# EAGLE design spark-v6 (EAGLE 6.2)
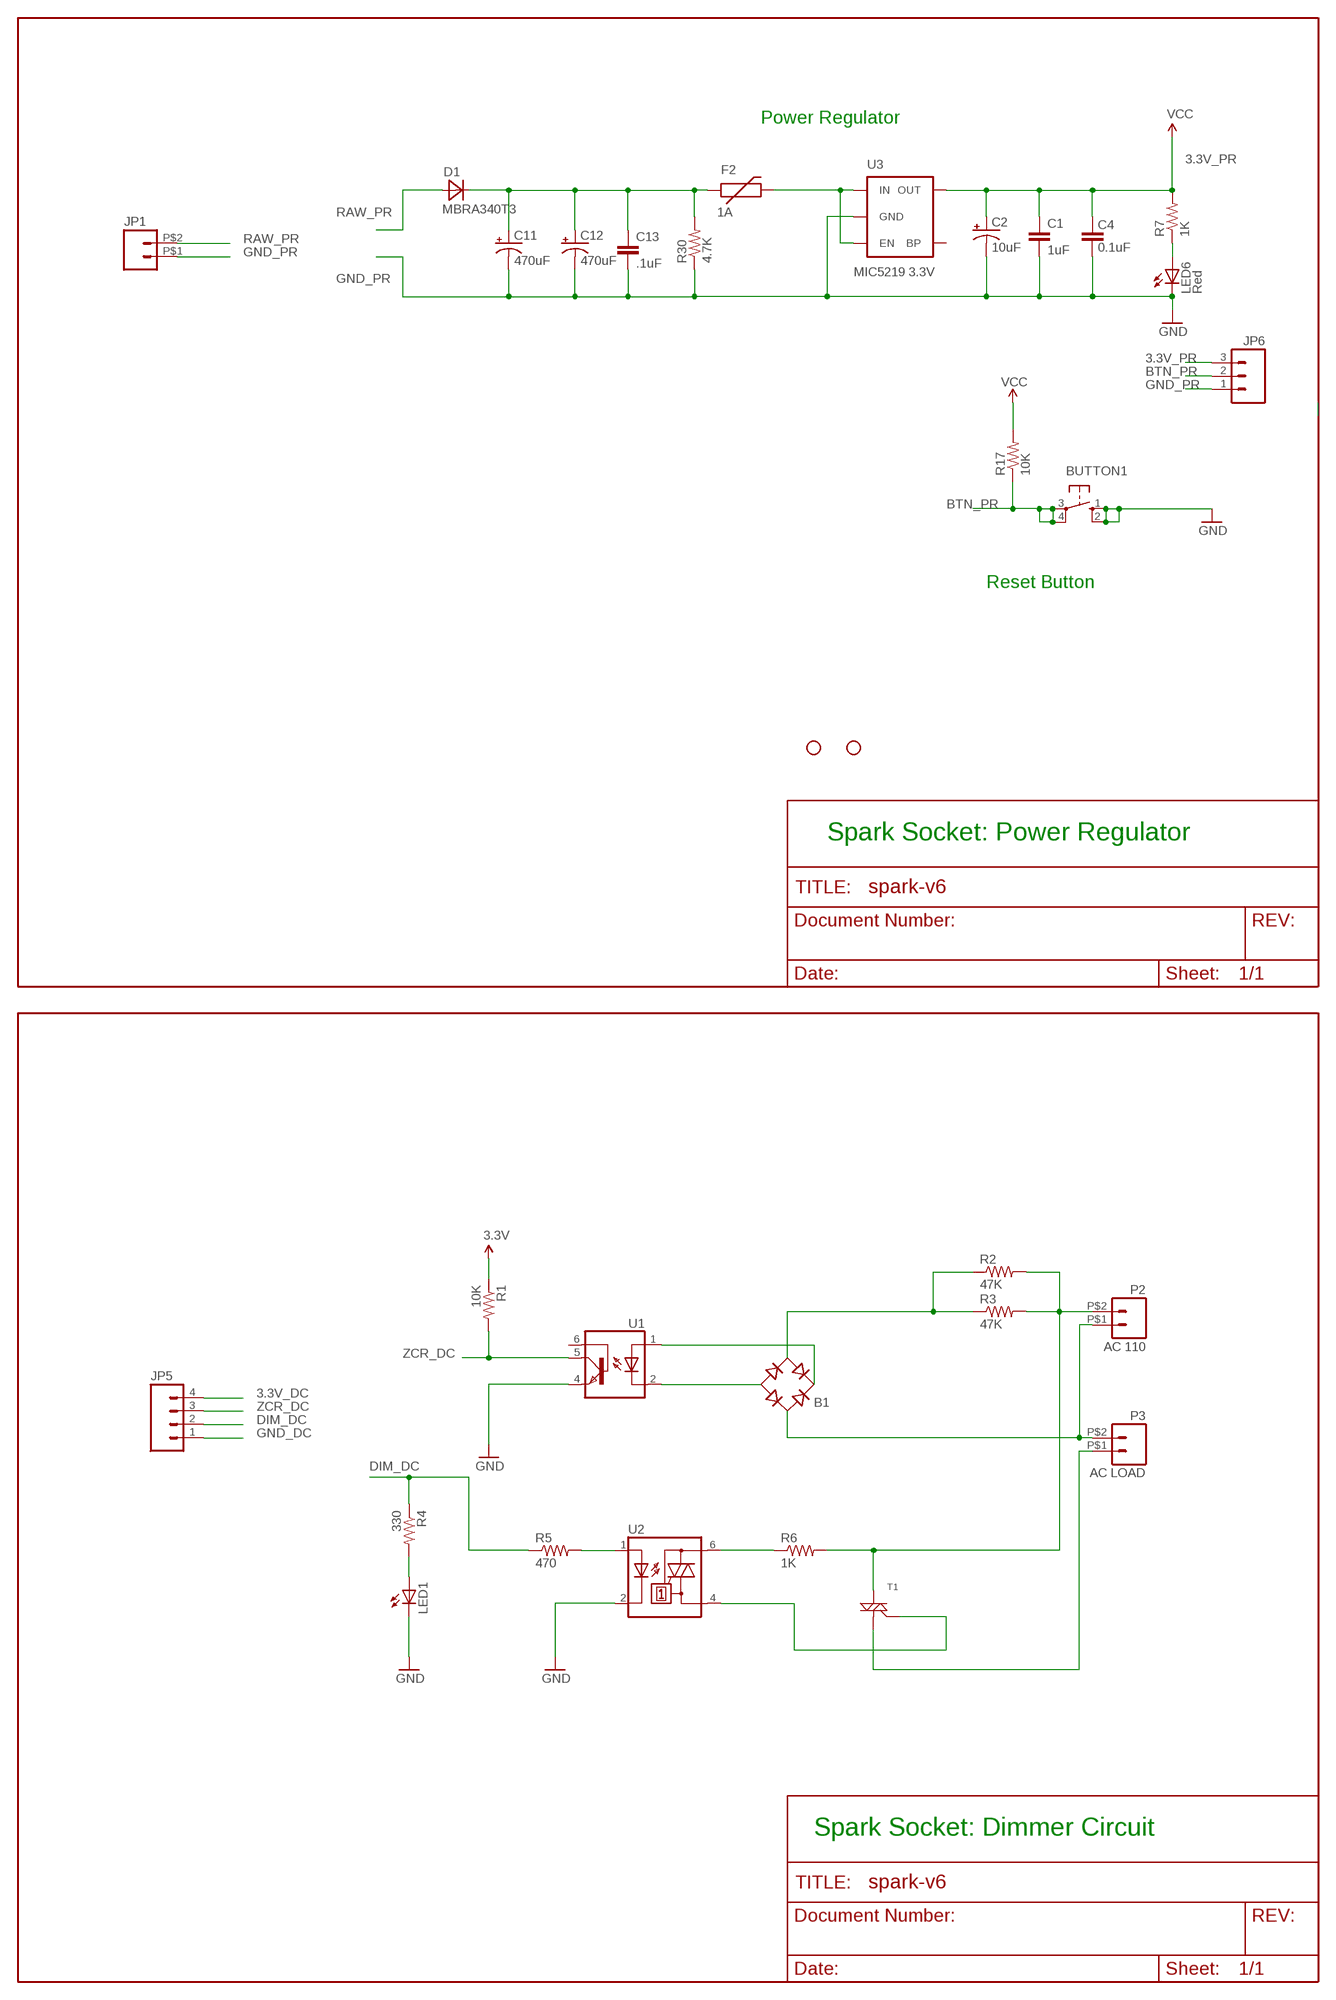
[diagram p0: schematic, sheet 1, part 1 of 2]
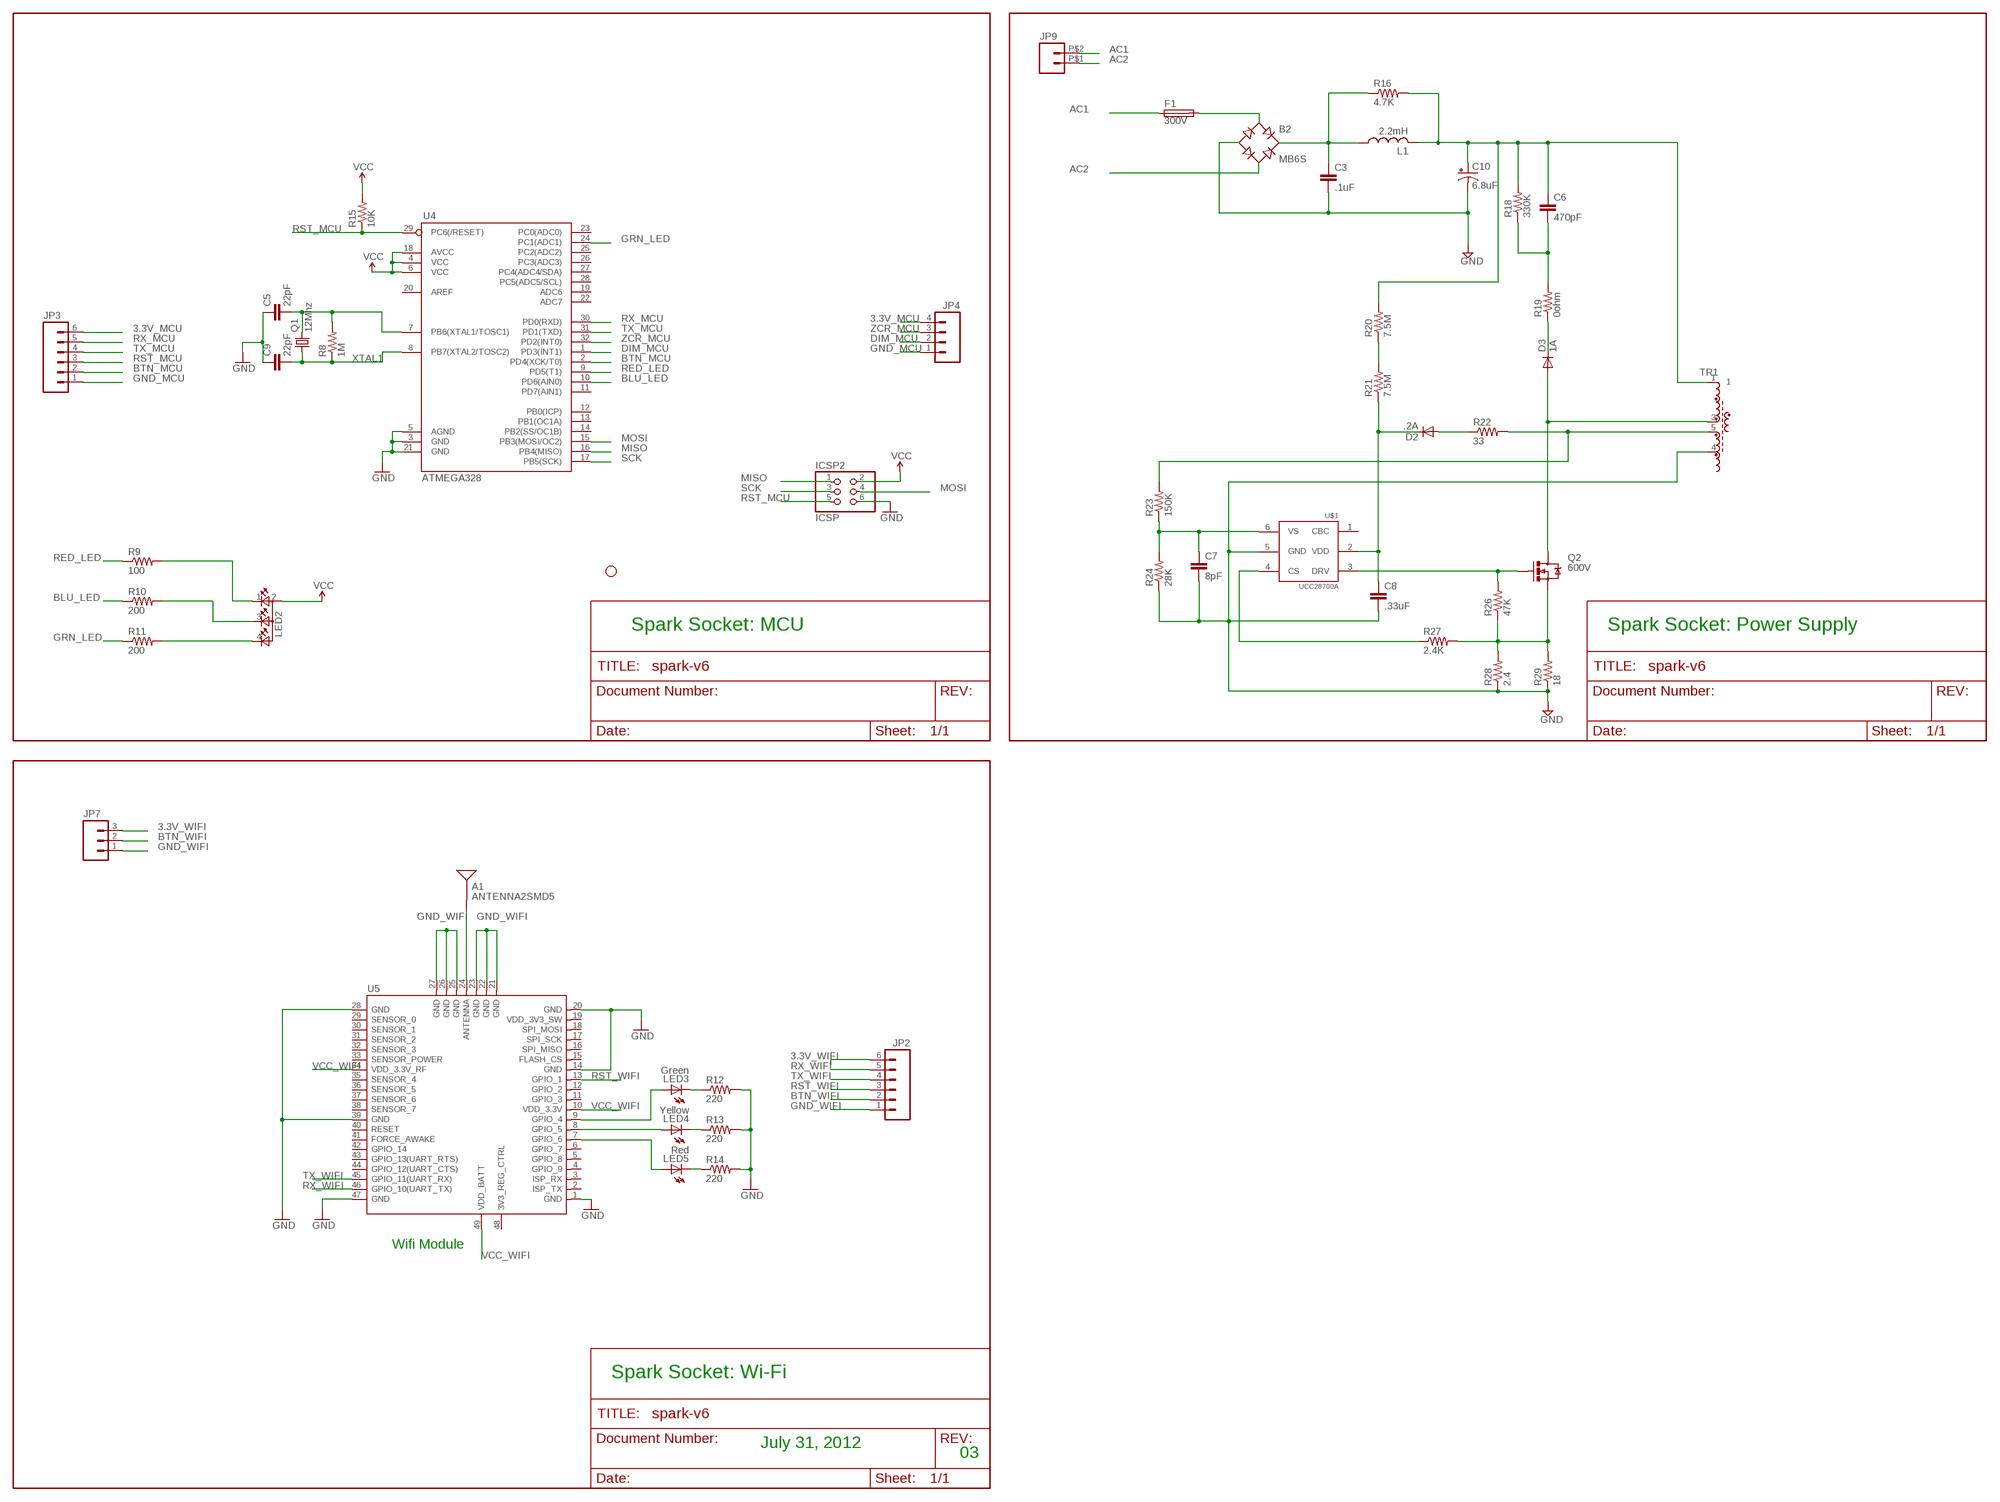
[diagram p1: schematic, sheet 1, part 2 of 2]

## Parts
A1  ANTENNA2SMD5  [ANTENNA-CHIP5]
B1  DF10S  [DFS]
B2  MB6S  [SOIC-4]
BUTTON1  10-XX  [B3F-10XX]
C1  1uF  CAP0603-CAP  [0603-CAP]
C2  10uF  CAP_POL1206  [EIA3216]
C3  .1uF  CAP1206  [1206]
C4  0.1uF  CAP0603-CAP  [0603-CAP]
C5  22pF  CAP0603-CAP  [0603-CAP]
C6  470pF  CAP1206  [1206]
C7  8pF  CAP0603-CAP  [0603-CAP]
C8  .33uF  CAP0603-CAP  [0603-CAP]
C9  22pF  CAP0603-CAP  [0603-CAP]
C10  6.8uF  CPOL-USE5-8.5  [E5-8,5]
C11  470uF  CAP_POL1206  [EIA3216]
C12  470uF  CAP_POL1206  [EIA3216]
C13  .1uF  CAP1206  [1206]
D1  MBRA340T3  [SMA]
D2  .2A  DIODESOD  [SOD-323]
D3  1A  DIODESMA  [SMA-DIODE]
F1  300V  TE5  [TE5]
F2  1A  PTCSMD  [PTC-1206]
ICSP2  ICSP  PINHD-2X3  [2X03]
JP1  M02PTH2  [1X02_BIG]
JP2  M06SIP  [1X06]
JP3  M06SIP  [1X06]
JP4  M04PTH  [1X04]
JP5  M04PTH  [1X04]
JP6  M03PTH  [1X03]
JP7  M03PTH  [1X03]
JP8  STAND-OFF  [STAND-OFF]
JP9  M02PTH2  [1X02_BIG]
JP10  STAND-OFF  [STAND-OFF]
JP11  STAND-OFF  [STAND-OFF]
L1  2.2mH  L-US0204V  [0204V]
LED1  LED0603  [LED-0603]
LED2  TOPLED-3PLCC  [P-LCC-4-3]
LED3  Green  LED0603  [LED-0603]
LED4  Yellow  LED0603  [LED-0603]
LED5  Red  LED0603  [LED-0603]
LED6  Red  LED0603  [LED-0603]
P2  AC 110  M02PTH2  [1X02_BIG]
P3  AC LOAD  M02PTH2  [1X02_BIG]
Q1  12Mhz  CRYSTALHC49UP  [HC49UP]
Q2  600V  MOSFET-NCHANNELPTH2  [TO220V]
R1  10K  RESISTOR0603-RES  [0603-RES]
R2  47K  RESISTOR0603-RES  [0603-RES]
R3  47K  RESISTOR0603-RES  [0603-RES]
R4  330  RESISTOR0603-RES  [0603-RES]
R5  470  RESISTOR0603-RES  [0603-RES]
R6  1K  RESISTOR0603-RES  [0603-RES]
R7  1K  RESISTOR0603-RES  [0603-RES]
R8  1M  RESISTOR0603-RES  [0603-RES]
R9  100  RESISTOR0603-RES  [0603-RES]
R10  200  RESISTOR0603-RES  [0603-RES]
R11  200  RESISTOR0603-RES  [0603-RES]
R12  220  RESISTOR0603-RES  [0603-RES]
R13  220  RESISTOR0603-RES  [0603-RES]
R14  220  RESISTOR0603-RES  [0603-RES]
R15  10K  RESISTOR0603-RES  [0603-RES]
R16  4.7K  RESISTOR0805-RES  [0805]
R17  10K  RESISTOR0603-RES  [0603-RES]
R18  330K  RESISTOR1206  [1206]
R19  0ohm  RESISTOR1206  [1206]
R20  7.5M  RESISTOR1206  [1206]
R21  7.5M  RESISTOR1206  [1206]
R22  33  RESISTOR0603-RES  [0603-RES]
R23  150K  RESISTOR0603-RES  [0603-RES]
R24  28K  RESISTOR0603-RES  [0603-RES]
R26  47K  RESISTOR0603-RES  [0603-RES]
R27  2.4K  RESISTOR0603-RES  [0603-RES]
R28  2.4  RESISTOR0603-RES  [0603-RES]
R29  18  RESISTOR0805-RES  [0805]
R30  4.7K  RESISTOR0603-RES  [0603-RES]
T1  TRIACSMD  [SOT223]
TR1  EMC13  [EMC13]
U1  4N25SM  [DIL6-SMD]
U2  MOC3031S  [DIL6-SMD]
U3  MIC5219 3.3V  V_REG_LDOSMD  [SOT23-5]
U4  ATMEGA328  ATMEGA168  [TQFP32-08]
U5  WIFI-RN-171  [49P-1.27-26.67X17.78]
U$1  UCC28700A  [DBV]

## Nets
3.3V_DC: JP5.4 R1.1 ; supply symbol labelled 3.3V
3.3V_MCU: ICSP2.2 JP3.6 JP4.4 LED2.2(A2) R15.2 U4.4(VCC) U4.6(VCC) U4.18(AVCC) ; supply symbol labelled VCC
3.3V_PR: C1.1 C2.A(+) C4.2 JP6.3 R7.2 R17.2 U3.5(OUT) ; supply symbol labelled VCC
3.3V_WIFI: JP2.6 JP7.3
AC1: F1.1 JP9.P$2
AC2: B2.~2(AC2) JP9.P$1
ASDF: C11.A(+) C12.A(+) C13.1 D1.C F2.1 R30.2
BLU_LED: R10.1 U4.10(PD6(AIN0))
BTN_MCU: JP3.2 U4.2(PD4(XCK/T0))
BTN_PR: BUTTON1.3(P) BUTTON1.4(P1) JP6.2 R17.1
BTN_WIFI: JP2.2 JP7.2
DIM_DC: JP5.2 R4.1 R5.1
DIM_MCU: JP4.2 U4.1(PD3(INT1))
GND: C7.2 C8.2 R24.1 R28.1 R29.1 TR1.4 U$1.5(GND)
GND_DC: JP5.1 LED1.C U1.4(EMI) U2.2(C) ; supply symbol labelled GND
GND_MCU: C5.1 C9.1 ICSP2.6 JP3.1 JP4.1 U4.3(GND) U4.5(AGND) U4.21(GND) ; supply symbol labelled GND
GND_POWER: B2.- C3.2 C10.- ; supply symbol labelled GND
GND_PR: BUTTON1.1(S) BUTTON1.2(S1) C1.2 C2.C(-) C4.1 C11.C(-) C12.C(-) C13.2 JP1.P$1 JP6.1 LED6.C R30.1 U3.2(GND) ; supply symbol labelled GND
GND_WIFI: JP2.1 JP7.1 R12.2 R13.2 R14.2 U5.1(GND) U5.14(GND) U5.20(GND) U5.21(GND) U5.22(GND) U5.23(GND) U5.25(GND) U5.26(GND) U5.27(GND) U5.28(GND) U5.39(GND) U5.47(GND) ; supply symbol labelled GND
GRN_LED: R11.1 U4.24(PC1(ADC1))
MISO: ICSP2.1 U4.16(PB4(MISO))
MOSI: ICSP2.4 U4.15(PB3(MOSI/OC2))
N$1: LED2.1(CRED) R9.2
N$2: LED6.A R7.1
N$3: F2.2 U3.1(IN) U3.3(EN)
N$4: B1.- U1.2(C)
N$5: B1.+ U1.1(A)
N$6: B1.AC2 R2.1 R3.1
N$7: P2.P$2 R2.2 R3.2 R6.2 T1.2(M2)
N$8: LED2.4(CGREEN) R11.2
N$9: R6.1 U2.6(A2)
N$10: T1.3(G) U2.4(A1)
N$11: P3.P$1 T1.1(M1)
N$12: B1.AC1 P2.P$1 P3.P$2
N$13: LED1.A R4.2
N$15: LED2.3(CBLUE) R10.2
N$16: R5.2 U2.1(A)
N$18: B2.~1(AC1) F1.2
N$19: LED3.A U5.9(GPIO_4)
N$20: LED3.C R12.1
N$21: LED4.C R13.1
N$22: LED5.C R14.1
N$23: LED4.A U5.8(GPIO_5)
N$24: LED5.A U5.7(GPIO_6)
N$25: A1.FEED(SIGNAL) U5.24(ANTENNA)
N$26: R20.1 R21.2
N$27: B2.+ C3.1 L1.1 R16.1
N$28: C6.1 C10.+ L1.2 R16.2 R18.2 R20.2 TR1.1
N$29: C6.2 R18.1 R19.2
N$30: D3.A Q2.2(D) TR1.3
N$31: C7.1 R23.1 R24.2 U$1.6(VS)
N$32: D3.C R19.1
N$34: D2.2(A) R22.1
N$35: R22.2 R23.2 TR1.5
N$36: C8.1 D2.1(C) R21.1 U$1.2(VDD)
N$37: R27.1 U$1.4(CS)
N$38: C5.2 Q1.2 R8.2 U4.7(PB6(XTAL1/TOSC1))
N$39: Q2.1(G) R26.2 U$1.3(DRV)
N$40: Q2.3(S) R26.1 R27.2 R28.2 R29.2
RAW_PR: D1.A JP1.P$2
RED_LED: R9.1 U4.9(PD5(T1))
RST_MCU: ICSP2.5 JP3.3 R15.1
RST_WIFI: JP2.3 U5.13(GPIO_1)
RX_MCU: JP3.5 U4.30(PD0(RXD))
RX_WIFI: JP2.5 U5.46(GPIO_10(UART_TX))
SCK: ICSP2.3 U4.17(PB5(SCK))
TX_MCU: JP3.4 U4.31(PD1(TXD))
TX_WIFI: JP2.4 U5.45(GPIO_11(UART_RX))
VCC_WIFI: U5.10(VDD_3.3V) U5.34(VDD_3.3V_RF) U5.49(VDD_BATT)
XTAL1: C9.2 Q1.1 R8.1
ZCR_DC: JP5.3 R1.2 U1.5(COL)
ZCR_MCU: JP4.3 U4.32(PD2(INT0))
Unconnected: U1.6(BAS) U3.4(BP) U4.8(PB7(XTAL2/TOSC2)) U4.11(PD7(AIN1)) U4.12(PB0(ICP)) U4.13(PB1(OC1A)) U4.14(PB2(SS/OC1B)) U4.19(ADC6) U4.20(AREF) U4.22(ADC7) U4.23(PC0(ADC0)) U4.25(PC2(ADC2)) U4.26(PC3(ADC3)) U4.27(PC4(ADC4/SDA)) U4.28(PC5(ADC5/SCL)) U4.29(PC6(/RESET)) U5.2(ISP_TX) U5.3(ISP_RX) U5.4(GPIO_9) U5.5(GPIO_8) U5.6(GPIO_7) U5.11(GPIO_3) U5.12(GPIO_2) U5.15(FLASH_CS) U5.16(SPI_MISO) U5.17(SPI_SCK) U5.18(SPI_MOSI) U5.19(VDD_3V3_SW) U5.29(SENSOR_0) U5.30(SENSOR_1) U5.31(SENSOR_2) U5.32(SENSOR_3) U5.33(SENSOR_POWER) U5.35(SENSOR_4) U5.36(SENSOR_5) U5.37(SENSOR_6) U5.38(SENSOR_7) U5.40(RESET) U5.41(FORCE_AWAKE) U5.42(GPIO_14) U5.43(GPIO_13(UART_RTS)) U5.44(GPIO_12(UART_CTS)) U5.48(3V3_REG_CTRL) U$1.1(CBC)

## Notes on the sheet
- Power Regulator
- Reset Button
- Spark Socket: Power Regulator | Spark Socket: MCU | Spark Socket: Power Supply
- Wifi Module
- Spark Socket: Dimmer Circuit | Spark Socket: Wi-Fi
- July 31, 2012
- 03

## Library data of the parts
A1 = SparkFun:ANTENNA2: Antenna
B1 = rectifier:DF*S: Surface Mount Glass Passivated Bridge Rectifiers Source: Source: Comchip Bridge Rectifiers DF005S-G thru DF10S-G.pdf
B2 = rectifier:MB*S: Bridge Rectifier Source: http://www.fairchildsemi.com/ds/MB/MB6S.pdf
BUTTON1 = switch-omron:10-XX: OMRON SWITCH; MPN: B3F-1000; OC_FARNELL: 176432; OC_NEWARK: 36M3542
C1 C3-C9 C13 = SparkFun:CAP: Capacitor
C2 C11 C12 = SparkFun:CAP_POL: Capacitor Polarized
C10 = adafruit:CPOL-US: POLARIZED CAPACITOR, American symbol
D1 = diode:MBRA340T3: Surface Mount Schottky Power Rectifier
D2 D3 = SparkFun:DIODE: Diode
F1 = fuse:TE5: FUSE; OC_FARNELL: unknown; OC_NEWARK: unknown
F2 = SparkFun:PTC: Resettable Fuse PTC
ICSP2 = pinhead:PINHD-2X3: PIN HEADER
JP1 JP9 P2 P3 = SparkFun:M02: Header 2
JP2 JP3 = SparkFun:M06: Header 6 Standard 6-pin 0.1" header. Use with straight break away headers (SKU : PRT-00116), right angle break away headers (PRT-00553), swiss pins (PRT-00743), machine pins (PRT-00117), and female headers (PRT-00115). Molex polarized connector foot print use with SKU : PRT-08094 with associated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
JP4 JP5 = SparkFun:M04: Header 4 Standard 4-pin 0.1" header. Use with straight break away headers (SKU : PRT-00116), right angle break away headers (PRT-00553), swiss pins (PRT-00743), machine pins (PRT-00117), and female headers (PRT-00115). Molex polarized connector foot print use with SKU : PRT-08231 with associated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
JP6 JP7 = SparkFun:M03: Header 3 Standard 3-pin 0.1" header. Use with straight break away headers (SKU : PRT-00116), right angle break away headers (PRT-00553), swiss pins (PRT-00743), machine pins (PRT-00117), and female headers (PRT-00115). Molex polarized connector foot print use with SKU : PRT-08232 with associated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
JP8 JP10 JP11 = SparkFun:STAND-OFF: Stand Off
L1 = rcl:L-US: INDUCTOR, American symbol
LED1 LED3-LED6 = SparkFun:LED: LEDs
LED2 = Spark:TOPLED-3: Cree CLVBA-FKA
Q1 = crystal:CRYSTAL: CRYSTAL; OC_FARNELL: unknown; OC_NEWARK: unknown
Q2 = SparkFun:MOSFET-NCHANNEL
R1-R24 R26-R30 = SparkFun:RESISTOR: Resistor
T1 = SparkFun:TRIAC
TR1 = Spark:EMC13: TRANSFORMER SMD toroidal-core transformer with 3 windings
U1 = optocoupler:4N*?M: General Purpose 6-Pin Phototransistor Optocouplers Source: http://www.fairchildsemi.com/ds/4N/4N35-M.pdf; MF: FAIRCHILD SEMICONDUCTOR; MPN: 4N25SM; OC_FARNELL: 1021152; OC_NEWARK: 34C2020
U2 = optocoupler:MOC30*: 6-Pin DIP Zero-Cross Optoisolators Triac Driver Output (250/400 Volt Peak) Source: http://www.fairchildsemi.com/ds/MO/MOC3043-M.pdf; MF: FAIRCHILD SEMICONDUCTOR; MPN: MOC3031SM; OC_FARNELL: unknown; OC_NEWARK: 34C1335
U3 = SparkFun:V_REG_LDO: Voltage Regulator LDO Standard 150mA LDO voltage regulator in SOT-23 layout. Micrel part MIC5205. BP (by-pass) pin is used to lower output noise with 470pF cap.
U4 = SparkFun:ATMEGA168
U5 = Module:WIFI-RN-171: WIFLY GSX 802.11 b/g wireless LAN Module
U$1 = Spark:UCC28700

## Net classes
2 gnd: width 0.203 mm, drill 0.559 mm, clearance 0.152 mm
3 usbvcc: width 0.203 mm, drill 0.61 mm, clearance 0.152 mm
4 aref: width 0.203 mm, drill 0.61 mm, clearance 0.152 mm

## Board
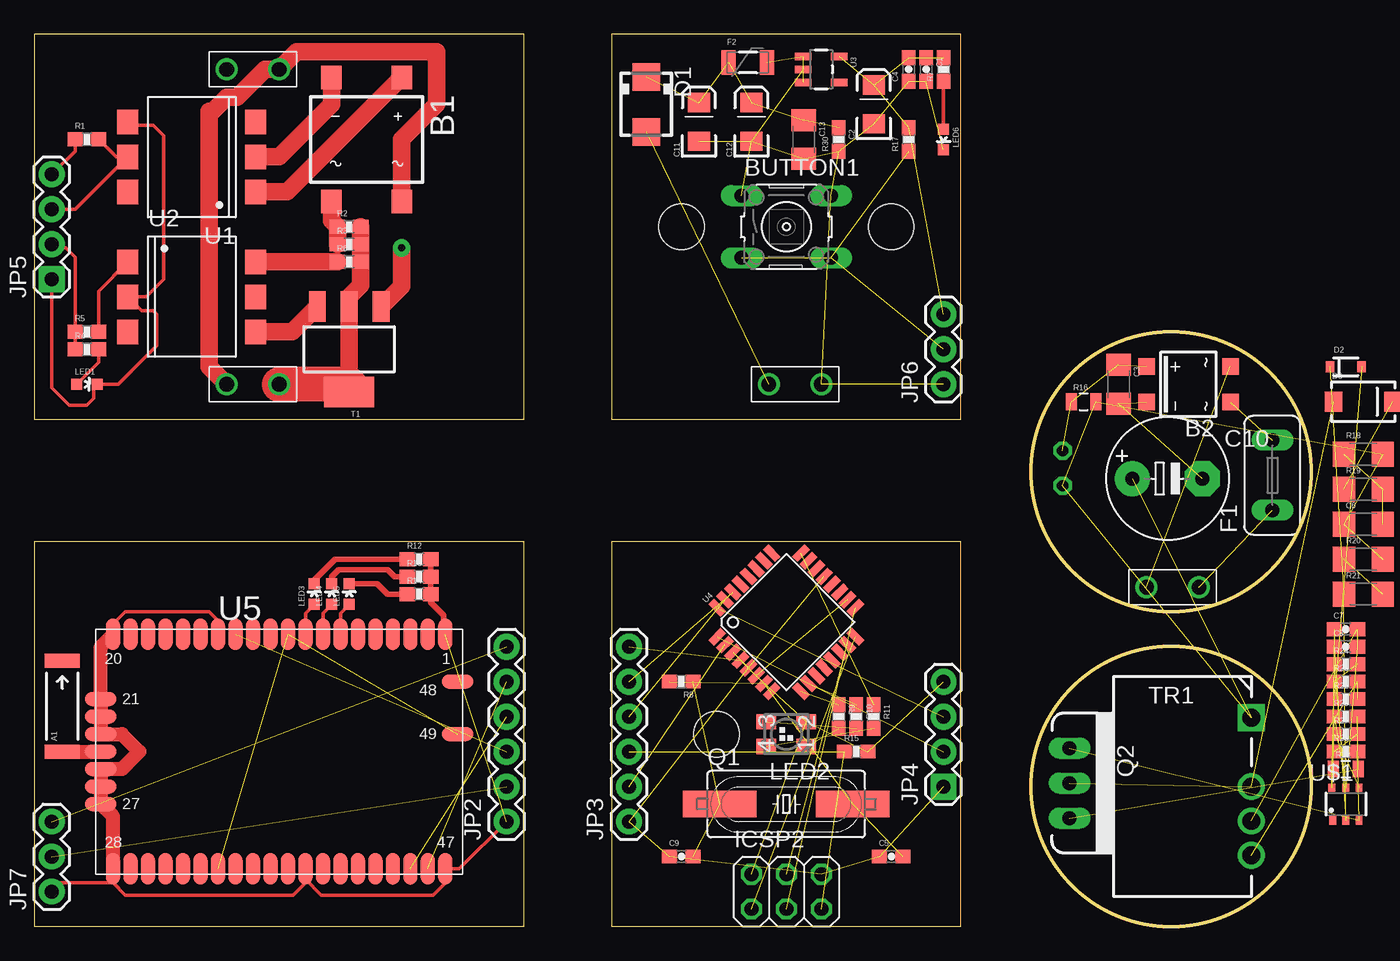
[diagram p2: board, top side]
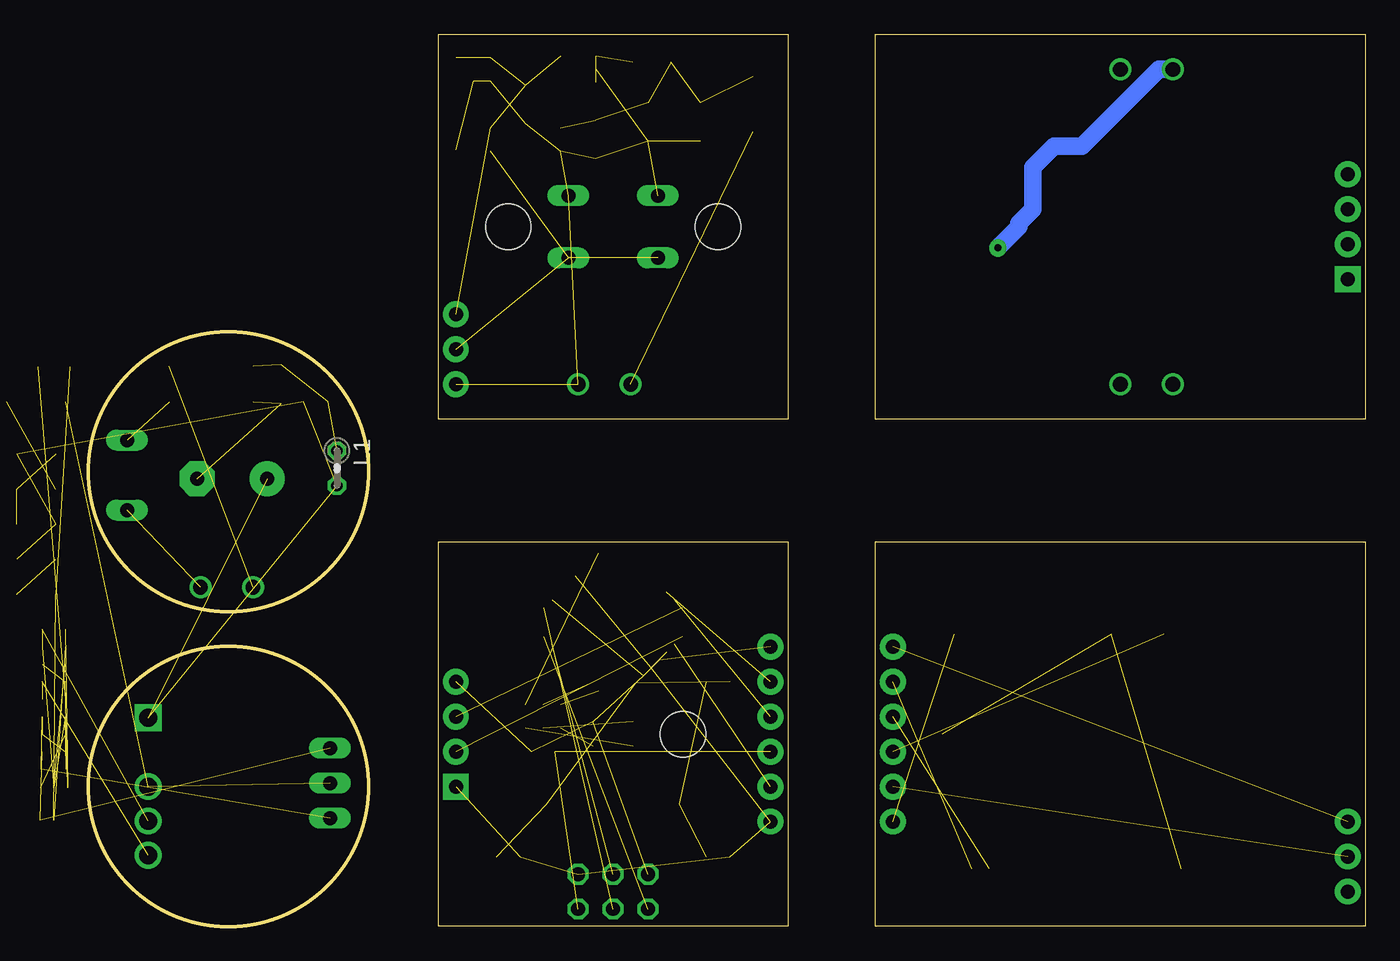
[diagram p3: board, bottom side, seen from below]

Size 92.71 x 64.77 mm. Coordinates in mm from the lower left corner, seen from the top.
Outline: 0,0 35.56,0 35.56,27.94 0,27.94 0,0
Outline: 41.91,0 67.31,0 67.31,27.94 41.91,27.94 41.91,0
Outline: 41.91,36.83 67.31,36.83 67.31,64.77 41.91,64.77 41.91,36.83
Outline: 0,36.83 35.56,36.83 35.56,64.77 0,64.77 0,36.83
Outline: circle at 82.55,10.16 radius 10.16
Outline: circle at 82.55,33.02 radius 10.16
Copper layers (1*16): Top 0.035mm / dielectric 1.5mm / Bottom 0.035mm
Design rules: minimum track width 10mil, minimum drill 24mil, track to track 8mil, track to pad 8mil, pad to pad 8mil, via to via 8mil, smd to smd 8mil, copper to edge 40mil, drill to drill 8mil, minimum pad ring 10mil, minimum via ring 8mil, stop-mask expansion 4mil, vias tented up to drill 0mil, thermal gap 10mil

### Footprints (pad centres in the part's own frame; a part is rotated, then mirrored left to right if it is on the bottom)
ANTENNA-CHIP5 = smd 1.016 x 2.54: FEED -3.302,0; NC 3.302,0
DFS = smd 1.5 x 1.7: + -2.55,-4.5; - 2.55,-4.5; AC1 -2.55,4.5; AC2 2.55,4.5
SOIC-4 = smd 1.2 x 1.2: + 1.3,3.05; - -1.3,3.05; ~1 -1.3,-3.05; ~2 1.3,-3.05
B3F-10XX = drill 1.016 long: 1 -3.251,2.261; 2 3.251,2.261; 3 -3.251,-2.261; 4 3.251,-2.261
0603-CAP = smd 1.1 x 1: 1 -0.85,0; 2 0.85,0
EIA3216 = smd 1.4 x 1.6: A 1.4,0; C -1.4,0
1206 = smd 1.6 x 1.8: 1 -1.4,0; 2 1.4,0
E5-8,5 = drill 1.016 pad 2.54: + -2.54,0 | drill 1.016 pad 2.54 octagon: - 2.54,0
SMA = smd 2 x 2: A 2,0; C -2,0
SOD-323 = smd 0.63 x 0.83: 1 -1.15,0; 2 1.15,0
SMA-DIODE = smd 1.27 x 1.47: A -2.15,0; C 2.15,0
TE5 = drill 1.016 long: 1 -2.54,0; 2 2.54,0
PTC-1206 = smd 1 x 1.8: 1 -1.4,0; 2 1.4,0
2X03 = drill 1.016 octagon: 1 -2.54,-1.27; 2 -2.54,1.27; 3 0,-1.27; 4 0,1.27; 5 2.54,-1.27; 6 2.54,1.27
1X02_BIG = drill 1.067: P$1 0,0; P$2 3.81,0
1X06 = drill 1.016 pad 1.88: 1 0,0; 2 2.54,0; 3 5.08,0; 4 7.62,0; 5 10.16,0; 6 12.7,0
1X04 = drill 1.016 pad 1.88 square: 1 0,0 | drill 1.016 pad 1.88: 2 2.54,0; 3 5.08,0; 4 7.62,0
1X03 = drill 1.016 pad 1.88: 1 0,0; 2 2.54,0; 3 5.08,0
STAND-OFF = hole 3.302: 0,0
0204V = drill 0.813 octagon: 1 -1.27,0; 2 1.27,0
LED-0603 = smd 0.8 x 0.8: A 0,-0.75; C 0,0.75
P-LCC-4-3 = smd 1.1 x 1.4: 1 -0.9,-1.45; 2 0.9,-1.45; 3 0.9,1.45; 4 -0.9,1.45
HC49UP = smd 5.334 x 1.93: 1 -4.826,0; 2 4.826,0
TO220V = drill 1.016 long: 1 -2.54,0; 2 0,0; 3 2.54,0
0603-RES = smd 1.1 x 1: 1 -0.85,0; 2 0.85,0
0805 = smd 0.8 x 1.2: 1 -0.9,0; 2 0.9,0
SOT223 = smd 1.219 x 2.235: 1 -2.311,-3.099; 2 0,-3.099; 3 2.311,-3.099 | smd 3.6 x 2.2: 4 0,3.099
EMC13 = drill 1.3 square: 1 0,5 | drill 1.3: 3 0,0; 4 0,-2.5; 5 0,-5
DIL6-SMD = smd 1.78 x 1.52: 1 -2.54,-4.645; 2 0,-4.645; 3 2.54,-4.645; 4 2.54,4.645; 5 0,4.645; 6 -2.54,4.645
SOT23-5 = smd 0.55 x 1.2: 1 -0.95,-1.3; 2 0,-1.3; 3 0.95,-1.3; 4 0.95,1.3; 5 -0.95,1.3
TQFP32-08 = smd 1.27 x 0.559: 1 -4.293,2.8; 2 -4.293,2; 3 -4.293,1.2; 4 -4.293,0.4; 5 -4.293,-0.4; 6 -4.293,-1.2; 7 -4.293,-2; 8 -4.293,-2.8; 17 4.293,-2.8; 18 4.293,-2; 19 4.293,-1.2; 20 4.293,-0.4; 21 4.293,0.4; 22 4.293,1.2; 23 4.293,2; 24 4.293,2.8 | smd 0.559 x 1.27: 9 -2.8,-4.293; 10 -2,-4.293; 11 -1.2,-4.293; 12 -0.4,-4.293; 13 0.4,-4.293; 14 1.2,-4.293; 15 2,-4.293; 16 2.8,-4.293; 25 2.8,4.293; 26 2,4.293; 27 1.2,4.293; 28 0.4,4.293; 29 -0.4,4.293; 30 -1.2,4.293; 31 -2,4.293; 32 -2.8,4.293
49P-1.27-26.67X17.78 = smd 1.016 x 2.286: 1 12.065,8.509; 2 10.795,8.509; 3 9.525,8.509; 4 8.255,8.509; 5 6.985,8.509; 6 5.715,8.509; 7 4.445,8.509; 8 3.175,8.509; 9 1.905,8.509; 10 0.635,8.509; 11 -0.635,8.509; 12 -1.905,8.509; 13 -3.175,8.509; 14 -4.445,8.509; 15 -5.715,8.509; 16 -6.985,8.509; 17 -8.255,8.509; 18 -9.525,8.509; 19 -10.795,8.509; 20 -12.065,8.509; 28 -12.065,-8.509; 29 -10.795,-8.509; 30 -9.525,-8.509; 31 -8.255,-8.509; 32 -6.985,-8.509; 33 -5.715,-8.509; 34 -4.445,-8.509; 35 -3.175,-8.509; 36 -1.905,-8.509; 37 -0.635,-8.509; 38 0.635,-8.509; 39 1.905,-8.509; 40 3.175,-8.509; 41 4.445,-8.509; 42 5.715,-8.509; 43 6.985,-8.509; 44 8.255,-8.509; 45 9.525,-8.509; 46 10.795,-8.509; 47 12.065,-8.509 | smd 2.286 x 1.016: 21 -12.954,3.81; 22 -12.954,2.54; 23 -12.954,1.27; 24 -12.954,0; 25 -12.954,-1.27; 26 -12.954,-2.54; 27 -12.954,-3.81; 48 12.954,5.08; 49 12.954,1.27
DBV = smd 0.5 x 0.6: 1 -0.96,-1.19; 2 0,-1.19; 3 0.96,-1.19; 4 0.96,1.19; 5 0,1.19; 6 -1.01,1.19

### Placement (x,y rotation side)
A1  2.03,16 90 top
B1  24.13,57.15 180 top
B2  83.82,39.37 90 top
BUTTON1  54.61,50.8 0 top
C1  64.77,62.23 270 top
C2  60.96,59.69 90 top
C3  78.74,39.37 270 top
C4  63.5,62.23 90 top
C5  62.23,5.08 0 top
C6  96.52,29.21 0 top
C7  95.25,21.59 0 top
C8  95.25,20.32 0 top
C9  46.99,5.08 0 top
C10  82.3,32.51 0 top
C11  48.26,58.42 90 top
C12  52.07,58.42 90 top
C13  55.88,57.15 270 top
D1  44.45,59.69 270 top
D2  95.25,40.64 0 top
D3  96.52,38.1 0 top
F1  89.92,32.77 90 top
F2  51.82,62.74 0 top
ICSP2  54.61,2.54 0 top
JP1  57.15,39.37 180 top
JP2  34.29,7.62 90 top
JP3  43.18,7.62 90 top
JP4  66.04,10.16 90 top
JP5  1.27,46.99 90 top
JP6  66.04,39.37 90 top
JP7  1.27,2.54 90 top
JP8  49.53,13.97 0 top
JP9  80.77,24.64 0 top
JP10  46.99,50.8 0 top
JP11  62.23,50.8 0 top
L1  74.68,33.27 270 bottom
LED1  3.81,39.37 270 top
LED2  54.61,13.97 90 top
LED3  20.32,24.13 0 top
LED4  21.59,24.13 0 top
LED5  22.86,24.13 0 top
LED6  66.04,57.15 180 top
P2  13.97,39.37 0 top
P3  13.97,62.23 0 top
Q1  54.61,8.89 0 top
Q2  75.18,10.41 270 top
R1  3.81,57.15 0 top
R2  22.86,50.8 0 top
R3  22.86,49.53 0 top
R4  3.81,41.91 0 top
R5  3.81,43.18 0 top
R6  22.86,48.26 0 top
R7  66.04,62.23 90 top
R8  46.99,17.78 180 top
R9  58.42,15.24 270 top
R10  59.69,15.24 270 top
R11  60.96,15.24 270 top
R12  27.94,26.67 0 top
R13  27.94,25.4 0 top
R14  27.94,24.13 0 top
R15  59.69,12.7 0 top
R16  76.2,38.1 0 top
R17  63.5,57.15 90 top
R18  96.52,34.29 0 top
R19  96.52,31.75 0 top
R20  96.52,26.67 0 top
R21  96.52,24.13 0 top
R22  95.25,16.51 0 top
R23  95.25,17.78 0 top
R24  95.25,19.05 0 top
R26  95.25,12.7 0 top
R27  95.25,13.97 0 top
R28  95.25,15.24 0 top
R29  95.25,11.43 0 top
R30  58.42,57.15 90 top
T1  22.86,41.91 180 top
TR1  88.39,10.16 0 top
U1  11.43,55.88 90 top
U2  11.43,45.72 270 top
U3  57.15,62.23 270 top
U4  54.61,22.1 45 top
U5  17.78,12.7 0 top
U$1  95.25,8.89 0 top

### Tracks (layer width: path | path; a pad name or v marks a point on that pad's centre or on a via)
3.3V_DC
  Top 0.254: R1.1 2.96,56.3 JP5.4
3.3V_MCU  (7 unrouted)
3.3V_PR  (6 unrouted)
3.3V_WIFI  (1 unrouted)
AC1  (1 unrouted)
AC2  (1 unrouted)
ASDF  (5 unrouted)
BLU_LED  (1 unrouted)
BTN_MCU  (1 unrouted)
BTN_PR  (3 unrouted)
BTN_WIFI  (1 unrouted)
DIM_DC
  Top 0.254: R4.1 R5.1 2.96,48.6 2.29,49.28 1.52,49.28 JP5.2
DIM_MCU  (1 unrouted)
GND  (6 unrouted)
GND_DC
  Top 0.254: U1.4 7.04,58.17 8.64,58.17 9.4,57.4 9.4,46.99 8.13,45.72 U2.2 7.8,44.7 8.64,44.7 8.89,44.45 8.89,42.16 6.1,39.37 LED1.C 4.32,39.13 4.32,38.35 3.81,37.85 2.54,37.85 1.27,39.12 JP5.1
GND_MCU  (7 unrouted)
GND_POWER  (2 unrouted)
GND_PR  (12 unrouted)
GND_WIFI  (1 unrouted)
  Top 0.254: U5.28 5.71,3.17 | 5.71,3.17 6.6,2.29 18.8,2.29 19.56,3.05 19.56,4.06 U5.39 19.68,3.43 20.83,2.29 28.96,2.29 29.97,3.3 29.97,4.06 U5.47 30.86,4.19 JP2.1 | 5.71,3.17 1.91,3.17 JP7.1 | U5.20 5.71,21.97 6.6,22.86 12.7,22.86 13.46,22.1 13.46,21.34 U5.14
  Top 0.406: R12.2 R13.2 R14.2 28.79,23.53 29.72,22.61 29.72,21.34 U5.1
  Top 1.016: U5.20 4.83,20.32 U5.21 U5.22 U5.23 6.35,13.97 7.62,12.7 6.35,11.43 U5.25 U5.26 U5.27 5.71,8 U5.28
GRN_LED  (1 unrouted)
MISO  (1 unrouted)
MOSI  (1 unrouted)
N$1  (1 unrouted)
N$2
  Top 0.254: R7.1 LED6.A
N$3  (2 unrouted)
N$4
  Top 1.27: U1.2 17.78,55.88 21.59,59.69 B1.-
N$5
  Top 1.27: U1.1 18.37,53.34 B1.+
N$6
  Top 1.27: B1.AC2 21.58,51.23 R2.1 R3.1
N$7
  Top 1.27: R2.2 R3.2 R6.2 23.71,46.57 22.86,45.72 T1.2 22.86,39.37
  Top 2.54: 22.86,39.37 P2.P$2
N$8  (1 unrouted)
N$9
  Top 1.27: R6.1 U2.6
N$10
  Top 1.27: U2.4 18.72,43.18 T1.3
N$11  (via drill 0.51 pad 1.27)
  Top 1.27: T1.1 25.2,45.01 26.67,46.48 v26.67,49.28
  Bottom 1.27: P3.P$1 14.99,62.23 20.57,56.64 22.61,56.64 24.13,55.12 24.13,52.07 25.15,51.05 25.15,50.8 v26.67,49.28
N$12
  Top 1.27: B1.AC1 26.68,57.16 29.21,59.69 29.21,63.5 19.05,63.5 P3.P$2 16.76,62.23 14.73,60.2 13.97,60.2 12.95,59.18 12.7,59.18 12.7,40.64 P2.P$1
N$13
  Top 0.254: R4.2 4.66,40.97 LED1.A
N$15  (1 unrouted)
N$16
  Top 0.254: R5.2 4.66,46.13 U2.1
N$18  (1 unrouted)
N$19
  Top 0.254: U5.9 19.68,22.75 LED3.A
N$20
  Top 0.406: LED3.C 20.32,25.15 21.84,26.67 R12.1
N$21
  Top 0.406: LED4.C 21.59,25.4 22.1,25.91 25.65,25.91 26.16,25.4 R13.1
N$22
  Top 0.406: LED5.C 24.9,24.88 25.65,24.13 R14.1
N$23
  Top 0.254: U5.8 20.95,22.75 LED4.A
N$24
  Top 0.254: U5.7 22.23,22.75 LED5.A
N$25
  Top 1.016: A1.FEED U5.24
N$26  (1 unrouted)
N$27  (3 unrouted)
N$28  (6 unrouted)
N$29  (2 unrouted)
N$30  (2 unrouted)
N$31  (3 unrouted)
N$32  (1 unrouted)
N$34  (1 unrouted)
N$35  (2 unrouted)
N$36  (3 unrouted)
N$37  (1 unrouted)
N$38  (3 unrouted)
N$39  (2 unrouted)
N$40  (4 unrouted)
RAW_PR  (1 unrouted)
RED_LED  (1 unrouted)
RST_MCU  (2 unrouted)
RST_WIFI  (1 unrouted)
RX_MCU  (1 unrouted)
RX_WIFI  (1 unrouted)
SCK  (1 unrouted)
TX_MCU  (1 unrouted)
TX_WIFI  (1 unrouted)
VCC_WIFI  (2 unrouted)
XTAL1  (2 unrouted)
ZCR_DC
  Top 0.254: R1.2 5.93,55.88 U1.5 2.98,52.07 JP5.3
ZCR_MCU  (1 unrouted)

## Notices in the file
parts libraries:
SparkFun: Licensing: CC v3.0 Share-Alike You are welcome to use this library for commercial purposes.
